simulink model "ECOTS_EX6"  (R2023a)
settings: Solver=ode23tb  StartTime=0.0  StopTime=meas.Time(end)  RelTol=1e-3
libraries: component_lib x33, slpidlib x2

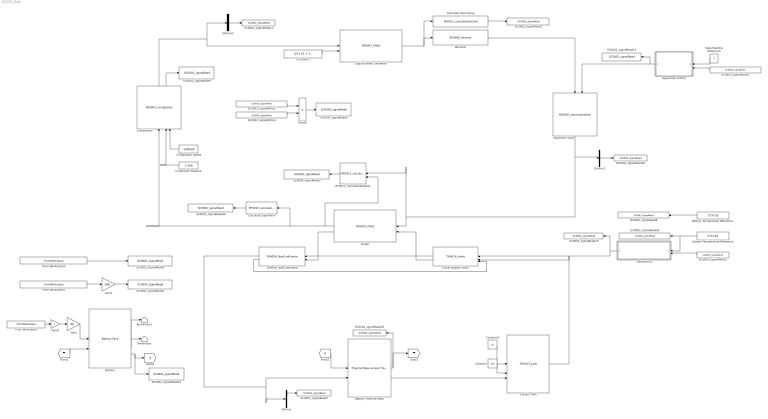
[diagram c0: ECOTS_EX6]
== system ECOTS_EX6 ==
  Battery : component_lib/Battery Pack  SOC_0=1  Nx=40  Ny=180
  Battery Temperature Reference : Constant  Value=273+25
  Battery Thermal Mass : component_lib/Thermal Mass & Heat Transfer  n=100  d=10e-3  L=4  m=40 * 180 * 0.048  cp=1040  T_0=273 + 25
  Calculate Subcooling : component_lib/Thermal Systems/RF0011_calculateSubCool
  Calculate Superheat : component_lib/Thermal Systems/RF0010_calculateSuperHeat
  Chiller : component_lib/Thermal Systems/RF0007_PHEX  N_ch=10  L=180e-3  B=65e-3  H=2e-3  t=0.3e-3  D_h=2.61e-3  N_nod=10
  Chiller Bypass Valve : component_lib/Thermal Systems/TH0014_valve  d=10e-2  dr=5e-2  C_d=0.9
  Compressor : component_lib/Thermal Systems/RF0003_compressor  V_disp=0.00017  N_ref=2000
  Compressor Speed : Constant  Value=1000/60
  Condenser Pressure : Constant  Value=1.3e6
  Constant : Constant  Value=2e5
  Constant1 : Constant  Value=[273.15 + 30; 1e5; 0.3]
  Constant2 : Constant  Value=0.1
  Coolant Tank : component_lib/Thermal Systems/TH0013_tank  V=5e-3  T0=273.15 + 25
  Coolant Temperature Reference : Constant  Value=273+20
  Demux : Demux  Outputs=3
  Demux1 : Demux  Outputs=3
  Demux2 : Demux  Outputs=3
  Divide : Product  Inputs=*/
  Expansion Valve : component_lib/Thermal Systems/RF0005_expansionValve  D=3*1.8e-3  p_min=50e3
  From Workspace : FromWorkspace  VariableName=[meas.Time, meas.Current]
  From Workspace1 : FromWorkspace  VariableName=[meas.Time, meas.Voltage]
  From Workspace2 : FromWorkspace  VariableName=[meas.Time, meas.Battery_Temp_degC + 273.15]
  Gain : Gain  Gain=40
  Gain1 : Gain  Gain=180
  Gain2 : Gain  Gain=-1
  Liquid-cooled Condenser : component_lib/Thermal Systems/RF0007_PHEX  N_ch=20  L=180e-3  B=65e-3  H=2e-3  t=0.3e-3  D_h=2.61e-3  N_nod=10
  RF0013_calculateHeatflow : component_lib/Thermal Systems/RF0013_calculateHeatflow
  Receiver : component_lib/Thermal Systems/RF0008_receiver  V=1e-3  h0=280e3  p0=1.6e6  p_gain=1e-2
  SC0002_signalRead1 : component_lib/Data & Control/SC0002_signalRead  SigName=condenserSubCooling
  SC0002_signalRead10 : component_lib/Data & Control/SC0002_signalRead  SigName=evaporatorPressure
  SC0002_signalRead11 : component_lib/Data & Control/SC0002_signalRead  SigName=condenserPressure
  SC0002_signalRead14 : component_lib/Data & Control/SC0002_signalRead  SigName=generatedHeat
  SC0002_signalRead15 : component_lib/Data & Control/SC0002_signalRead  SigName=expansionValve
  SC0002_signalRead19 : component_lib/Data & Control/SC0002_signalRead  SigName=chillerBypassValve
  SC0002_signalRead2 : component_lib/Data & Control/SC0002_signalRead  SigName=evaporatorCooling
  SC0002_signalRead21 : component_lib/Data & Control/SC0002_signalRead  SigName=coolantTemperatureReference
  SC0002_signalRead22 : component_lib/Data & Control/SC0002_signalRead  SigName=batteryTemperature
  SC0002_signalRead3 : component_lib/Data & Control/SC0002_signalRead  SigName=measuredBatteryVoltage
  SC0002_signalRead4 : component_lib/Data & Control/SC0002_signalRead  SigName=measuredBatteryTemperature
  SC0002_signalRead40 : component_lib/Data & Control/SC0002_signalRead  SigName=evaporatorSuperheat
  SC0002_signalRead5 : component_lib/Data & Control/SC0002_signalRead  SigName=COOP
  SC0002_signalRead7 : component_lib/Data & Control/SC0002_signalRead  SigName=coolantTemperature
  SC0002_signalRead8 : component_lib/Data & Control/SC0002_signalRead  SigName=batteryTemperatureReference
  SC0002_signalRead9 : component_lib/Data & Control/SC0002_signalRead  SigName=compressorPower
  SC0003_signalWrite1 : component_lib/Data & Control/SC0003_signalWrite  SigName=evaporatorCooling
  SC0003_signalWrite2 : component_lib/Data & Control/SC0003_signalWrite  SigName=evaporatorSuperheat
  SC0003_signalWrite3 : component_lib/Data & Control/SC0003_signalWrite  SigName=coolantTemperature
  SC0003_signalWrite4 : component_lib/Data & Control/SC0003_signalWrite  SigName=compressorPower
  Subsystem1 : Subsystem
  Superheat Control : Subsystem
  Superheating Reference : Constant  Value=5
  TH0006_flowConfluence : component_lib/Thermal Systems/TH0006_flowConfluence  gain=0.01
  Terminator : Terminator
  Terminator1 : Terminator
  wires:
  Calculate Superheat/1 -> SC0002_signalRead40/1
  Compressor Speed/1 -> Compressor/3
  Compressor/2 -> SC0002_signalRead9/1
  Liquid-cooled Condenser/1 -> Calculate Subcooling/1, Receiver/1
  Receiver/1 -> Expansion Valve/1
  Constant1/1 -> Liquid-cooled Condenser/2
  Calculate Subcooling/1 -> SC0002_signalRead1/1
  Superheating Reference/1 -> Superheat Control/1(T_ref [K])
  SC0003_signalWrite2/1 -> Superheat Control/2(T [K])
  Chiller/1 -> RF0013_calculateHeatflow/2, Compressor/1, Calculate Superheat/1
  Expansion Valve/1 -> RF0013_calculateHeatflow/1, Chiller/1, Demux1/1
  Battery/1 -> Terminator1/1
  [Q] -> Battery Thermal Mass/1
  Battery/2 -> Terminator/1
  Battery/3 -> SC0002_signalRead14/1, [Q]
  Battery Thermal Mass/1 -> [T], SC0002_signalRead22/1
  [T] -> Battery/2
  Constant/1 -> Coolant Tank/2
  Subsystem1/1(cv [-]) -> Chiller Bypass Valve/1, SC0002_signalRead19/1
  Coolant Temperature Reference/1 -> Subsystem1/1(T_ref [K]), SC0002_signalRead21/1
  SC0003_signalWrite3/1 -> Subsystem1/2(T [K])
  RF0013_calculateHeatflow/1 -> SC0002_signalRead2/1
  SC0003_signalWrite4/1 -> Divide/2
  SC0003_signalWrite1/1 -> Divide/1
  Divide/1 -> SC0002_signalRead5/1
  From Workspace1/1 -> Gain1/1
  From Workspace2/1 -> SC0002_signalRead4/1
  Gain1/1 -> SC0002_signalRead3/1
  Gain/1 -> Battery/1
  From Workspace/1 -> Gain2/1
  Gain2/1 -> Gain/1
  Condenser Pressure/1 -> Compressor/2
  Demux/1 -> SC0002_signalRead7/1
  Compressor/1 -> Demux2/1, Liquid-cooled Condenser/1
  Demux2/2 -> SC0002_signalRead11/1
  Chiller Bypass Valve/1 -> TH0006_flowConfluence/1
  Chiller Bypass Valve/2 -> Chiller/2
  Chiller/2 -> TH0006_flowConfluence/2
  TH0006_flowConfluence/1 -> Battery Thermal Mass/2, Demux/1
  TH0006_flowConfluence/2 -> Chiller Bypass Valve/3
  Coolant Tank/1 -> Chiller Bypass Valve/2
  Superheat Control/1(EXV [-]) -> Expansion Valve/2, SC0002_signalRead15/1
  Demux1/2 -> SC0002_signalRead10/1
  Constant2/1 -> Coolant Tank/1
  Battery Thermal Mass/2 -> Coolant Tank/3
  Battery Temperature Reference/1 -> SC0002_signalRead8/1

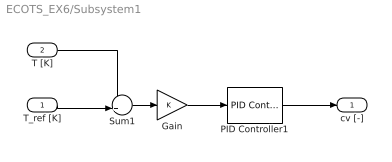
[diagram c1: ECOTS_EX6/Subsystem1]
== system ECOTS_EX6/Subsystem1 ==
  T_ref [K] : Inport
  T [K] : Inport  Port=2
  Gain : Gain
  PID Controller1 : slpidlib/PID Controller  Controller=PI  Form=Parallel  TimeDomain=Continuous-time  UseExternalTs=off  SampleTime=-1  IntegratorMethod=Forward Euler  FilterMethod=Forward Euler  ControllerParametersSource=internal  P=1e-1  I=1e-3  UseKiTs=off  D=0  N=100  UseFilter=on  TunerSelectOption=Transfer Function Based (PID Tuner App)  ZeroCross=off  InitialConditionSource=internal  InitialConditionForIntegrator=0.5  InitialConditionForFilter=0.5  DifferentiatorICPrevScaledInput=0  ExternalReset=none  TrackingMode=off  Kt=1  LimitOutput=on  SatLimitsSource=internal  UpperSaturationLimit=1  LowerSaturationLimit=0  LinearizeAsGain=on  AntiWindupMode=back-calculation  Kb=1  LimitIntegrator=off  UpperIntegratorSaturationLimit=inf  LowerIntegratorSaturationLimit=-inf  POutMin=[]  POutMax=[]  IOutMin=[]  IOutMax=[]  DOutMin=[]  DOutMax=[]  NOutMin=[]  NOutMax=[]  SumOutMin=[]  SumOutMax=[]  SaturationOutMin=[]  SaturationOutMax=[]  PParamMin=[]  PParamMax=[]  IParamMin=[]  IParamMax=[]  DParamMin=[]  DParamMax=[]  NParamMin=[]  NParamMax=[]  KbParamMin=[]  KbParamMax=[]  KtParamMin=[]  KtParamMax=[]  KbOutMin=[]  KbOutMax=[]  KtOutMin=[]  KtOutMax=[]  IntegratorOutMin=[]  IntegratorOutMax=[]  FilterOutMin=[]  FilterOutMax=[]  SumI1OutMin=[]  SumI1OutMax=[]  SumI2OutMin=[]  SumI2OutMax=[]  SumI3OutMin=[]  SumI3OutMax=[]  SumI4OutMin=[]  SumI4OutMax=[]  SumDOutMin=[]  SumDOutMax=[]  DifferentiatorOutMin=[]  DifferentiatorOutMax=[]  FilterDiffOutCoefMin=[]  FilterDiffOutCoefMax=[]  ReciprocalOutMin=[]  ReciprocalOutMax=[]  SumDenOutMin=[]  SumDenOutMax=[]  SumNumOutMin=[]  SumNumOutMax=[]  DivideOutMin=[]  DivideOutMax=[]  UdiffTsProdOutMin=[]  UdiffTsProdOutMax=[]  NTsProdOutMin=[]  NTsProdOutMax=[]  UintegralTsProdOutMin=[]  UintegralTsProdOutMax=[]  UngainTsProdOutMin=[]  UngainTsProdOutMax=[]  ClampingZeroOutDataTypeStr=Inherit: Inherit via back propagation  ClampingZeroOutMin=[]  ClampingZeroOutMax=[]  FilterDenConstantOutDataTypeStr=Inherit: Inherit via back propagation  FilterDenConstantOutMin=[]  FilterDenConstantOutMax=[]  PCopyOutDataTypeStr=Inherit: Inherit via back propagation  PCopyOutMin=[]  PCopyOutMax=[]  NCopyOutDataTypeStr=Inherit: Inherit via back propagation  NCopyOutMin=[]  NCopyOutMax=[]  IntegratorContinuousStateAttributes=''  IntegratorStateMustResolveToSignalObject=off  IntegratorRTWStateStorageClass=Auto  FilterContinuousStateAttributes=''  FilterStateMustResolveToSignalObject=off  FilterRTWStateStorageClass=Auto  ParallelPVariant=InternalParameters  IdealPVariant=Disabled  IVariant=InternalParameters  DVariant=Disabled  IntegratorVariant=Continuous  SatVariant=Enabled  AWVariant=BackCalculation  PCopyVariant=Disabled  TRVariant=Disabled  FdbkBlocksVariant=Forward  IdealPFdbkVariant=Disabled  SatFdbkVariant=Disabled  DerivativeFilterVariant=Disabled  NVariant=Disabled  NCopyVariant=Disabled_SignalSpec  FilterICVariant=Disabled  IntegratorICVariant=InternalICs  ExternalResetVariant=Disabled  TRSumVariant=Passthrough  SumFdbkVariant=Disabled  SumVariant=Sum_PI  TsampFilterVariant=InternalTs  TsampNgainVariant=Passthrough  TsampIntegralVariant=Disabled_SignalSpec  ExternalSaturationOutDataTypeStr=Inherit: Same as second input
  Sum1 : Sum  Inputs=-+|
  cv [-] : Outport
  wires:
  T [K]/1 -> Sum1/1
  Gain/1 -> PID Controller1/1
  Sum1/1 -> Gain/1
  PID Controller1/1 -> cv [-]/1
  T_ref [K]/1 -> Sum1/2

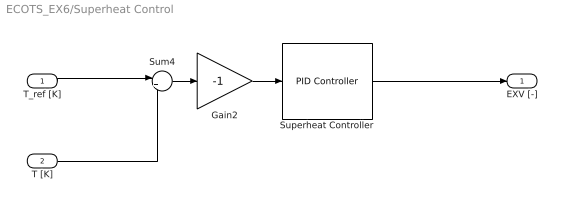
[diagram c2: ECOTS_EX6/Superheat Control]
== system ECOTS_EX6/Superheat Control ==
  T_ref [K] : Inport
  T [K] : Inport  Port=2
  Gain2 : Gain  Gain=-1
  Sum4 : Sum  Inputs=|+-
  Superheat Controller : slpidlib/PID Controller  Controller=PI  Form=Parallel  TimeDomain=Continuous-time  UseExternalTs=off  SampleTime=-1  IntegratorMethod=Forward Euler  FilterMethod=Forward Euler  ControllerParametersSource=internal  P=1e-3  I=1e-3  UseKiTs=off  D=0  N=100  UseFilter=on  TunerSelectOption=Transfer Function Based (PID Tuner App)  InitialConditionSource=internal  InitialConditionForIntegrator=0.3  InitialConditionForFilter=0  DifferentiatorICPrevScaledInput=0  ExternalReset=none  TrackingMode=off  Kt=1  LimitOutput=on  SatLimitsSource=internal  UpperSaturationLimit=0.999  LowerSaturationLimit=0.001  LinearizeAsGain=on  AntiWindupMode=back-calculation  Kb=1  LimitIntegrator=off  UpperIntegratorSaturationLimit=inf  LowerIntegratorSaturationLimit=-inf  POutMin=[]  POutMax=[]  IOutMin=[]  IOutMax=[]  DOutMin=[]  DOutMax=[]  NOutMin=[]  NOutMax=[]  SumOutMin=[]  SumOutMax=[]  SaturationOutMin=[]  SaturationOutMax=[]  PParamMin=[]  PParamMax=[]  IParamMin=[]  IParamMax=[]  DParamMin=[]  DParamMax=[]  NParamMin=[]  NParamMax=[]  KbParamMin=[]  KbParamMax=[]  KtParamMin=[]  KtParamMax=[]  KbOutMin=[]  KbOutMax=[]  KtOutMin=[]  KtOutMax=[]  IntegratorOutMin=[]  IntegratorOutMax=[]  FilterOutMin=[]  FilterOutMax=[]  SumI1OutMin=[]  SumI1OutMax=[]  SumI2OutMin=[]  SumI2OutMax=[]  SumI3OutMin=[]  SumI3OutMax=[]  SumI4OutMin=[]  SumI4OutMax=[]  SumDOutMin=[]  SumDOutMax=[]  DifferentiatorOutMin=[]  DifferentiatorOutMax=[]  FilterDiffOutCoefMin=[]  FilterDiffOutCoefMax=[]  ReciprocalOutMin=[]  ReciprocalOutMax=[]  SumDenOutMin=[]  SumDenOutMax=[]  SumNumOutMin=[]  SumNumOutMax=[]  DivideOutMin=[]  DivideOutMax=[]  UdiffTsProdOutMin=[]  UdiffTsProdOutMax=[]  NTsProdOutMin=[]  NTsProdOutMax=[]  UintegralTsProdOutMin=[]  UintegralTsProdOutMax=[]  UngainTsProdOutMin=[]  UngainTsProdOutMax=[]  ClampingZeroOutDataTypeStr=Inherit: Inherit via back propagation  ClampingZeroOutMin=[]  ClampingZeroOutMax=[]  FilterDenConstantOutDataTypeStr=Inherit: Inherit via back propagation  FilterDenConstantOutMin=[]  FilterDenConstantOutMax=[]  PCopyOutDataTypeStr=Inherit: Inherit via back propagation  PCopyOutMin=[]  PCopyOutMax=[]  NCopyOutDataTypeStr=Inherit: Inherit via back propagation  NCopyOutMin=[]  NCopyOutMax=[]  IntegratorContinuousStateAttributes=''  IntegratorStateMustResolveToSignalObject=off  IntegratorRTWStateStorageClass=Auto  FilterContinuousStateAttributes=''  FilterStateMustResolveToSignalObject=off  FilterRTWStateStorageClass=Auto  ParallelPVariant=InternalParameters  IdealPVariant=Disabled  IVariant=InternalParameters  DVariant=Disabled  IntegratorVariant=Continuous  SatVariant=Enabled  AWVariant=BackCalculation  PCopyVariant=Disabled  TRVariant=Disabled  FdbkBlocksVariant=Forward  IdealPFdbkVariant=Disabled  SatFdbkVariant=Disabled  DerivativeFilterVariant=Disabled  NVariant=Disabled  NCopyVariant=Disabled_SignalSpec  FilterICVariant=Disabled  IntegratorICVariant=InternalICs  ExternalResetVariant=Disabled  TRSumVariant=Passthrough  SumFdbkVariant=Disabled  SumVariant=Sum_PI  TsampFilterVariant=InternalTs  TsampNgainVariant=Passthrough  TsampIntegralVariant=Disabled_SignalSpec  ExternalSaturationOutDataTypeStr=Inherit: Same as second input
  EXV [-] : Outport
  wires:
  Sum4/1 -> Gain2/1
  T_ref [K]/1 -> Sum4/1
  T [K]/1 -> Sum4/2
  Gain2/1 -> Superheat Controller/1
  Superheat Controller/1 -> EXV [-]/1
